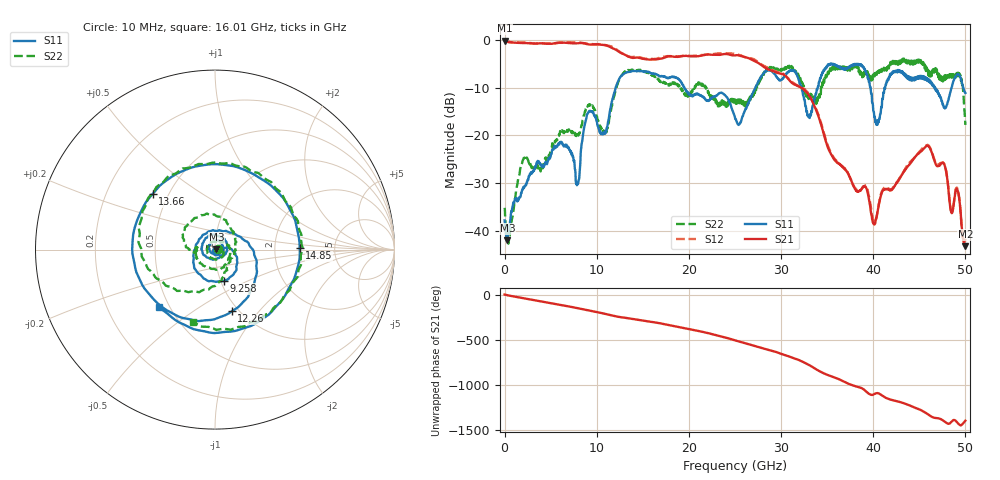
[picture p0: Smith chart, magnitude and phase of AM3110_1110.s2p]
# Hz S DB R 50.0
!freq dBS11 angS11 dBS21 angS21 dBS12 angS12 dBS22 angS22
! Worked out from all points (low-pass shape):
!   1601 points, 10 MHz to 50 GHz, reference 50 ohm
!   highest |S21| = -0.07 dB at 10 MHz (marker M1); lowest = -43.3 dB at 50 GHz (marker M2)
!   |S21| within 3 dB of the highest: start of sweep to 13.07 GHz; 23.37 GHz to 24.51 GHz (1.137 GHz wide, 4.75 % of centre)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
!   lowest |S11| = -42.1 dB at 322.4 MHz (marker M3), VSWR 1.02, Z = 50.8 + j0.201 ohm
!   |S11| at or under -10 dB: start of sweep to 12.05 GHz; 19.53 GHz to 27.2 GHz (7.675 GHz wide, 32.8 % of centre); 46.73 GHz to 48.5 GHz (1.774 GHz wide, 3.73 % of centre)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
!   |S22| runs from -42.8 to -3.9 dB; largest |S21 - S12| = 0.032
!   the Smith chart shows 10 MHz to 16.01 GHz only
!   S11 on the Smith chart (normalised r, x): 10 MHz: 1.02, -0.02; 9.258 GHz: 1.03, -0.37; 12.26 GHz: 0.93, -0.73; 13.66 GHz: 0.41, +0.32; 14.85 GHz: 2.79, +0.05; 16.01 GHz: 0.44, -0.35
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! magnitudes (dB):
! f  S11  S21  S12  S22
! 10 MHz  -37.9  -0.1  -0.1  -35.2
! 322.4 MHz  -42.1  -0.4  -0.3  -42.4
! 2.01 GHz  -31.0  -0.6  -0.5  -25.2
! 8.352 GHz  -22.0  -0.6  -0.5  -17.8
! 9.258 GHz  -14.9  -0.9  -0.8  -13.8
! 10.95 GHz  -19.5  -1.0  -1.0  -19.8
! 12.26 GHz  -9.0  -2.2  -2.1  -9.3
! 13.66 GHz  -6.6  -3.6  -3.5  -6.3
! 14.85 GHz  -6.5  -3.8  -3.7  -6.2
! 16.01 GHz  -7.0  -4.1  -3.9  -7.5
! 16.69 GHz  -7.4  -4.0  -3.8  -8.2
! 25 GHz  -16.3  -3.2  -2.9  -12.8
! 28.66 GHz  -6.2  -6.2  -5.9  -5.7
! 33.35 GHz  -15.0  -12.7  -12.5  -12.5
! 34.97 GHz  -5.4  -21.9  -21.6  -6.9
! 38.25 GHz  -5.0  -31.9  -31.6  -5.3
! 40.06 GHz  -15.0  -38.6  -38.1  -7.1
! 41.69 GHz  -7.9  -31.4  -31.2  -6.0
! 45.97 GHz  -8.2  -22.3  -22.1  -7.4
! 47.78 GHz  -14.3  -26.5  -26.4  -7.9
! 49.34 GHz  -7.4  -33.5  -33.3  -7.0
! 50 GHz  -11.1  -43.3  -41.8  -17.8
